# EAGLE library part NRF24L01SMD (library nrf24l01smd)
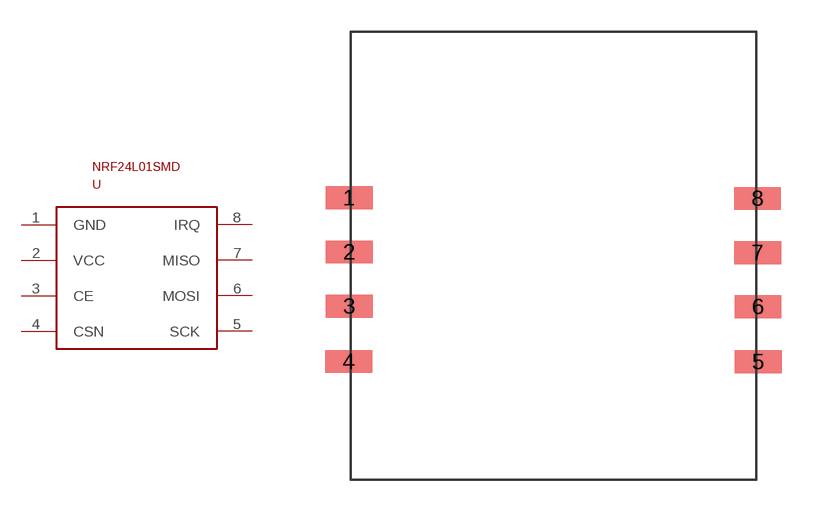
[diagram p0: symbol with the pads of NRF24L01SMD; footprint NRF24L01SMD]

Designator prefix -

## NRF24L01SMD  [NRF24L01SMD]
1  GND
2  VCC
3  CE
4  CSN
5  SCK
6  MOSI
7  MISO
8  IRQ

## Footprint NRF24L01SMD (pad centres in mm)
smd 2.184 x 1.067: 1 0,0; 2 0,-2.54; 3 0,-5.08; 4 -0.022,-7.677; 5 19.172,-7.686; 6 19.167,-5.102; 7 19.151,-2.57; 8 19.142,-0.027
